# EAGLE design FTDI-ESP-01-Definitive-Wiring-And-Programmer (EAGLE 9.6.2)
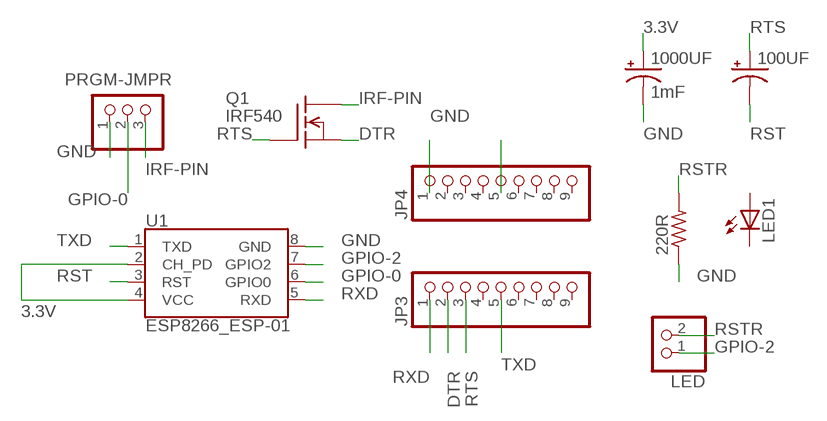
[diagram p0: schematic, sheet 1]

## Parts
100UF  CPOL-USE3.5-8  [E3,5-8]
220R  R-US_0207/2V  [0207/2V]
1000UF  1mF  1000UF-RADIAL-5MM-25V-20%  [CPOL-RADIAL-5MM-10MM]
JP3  PINHD-1X9  [1X09]
JP4  PINHD-1X9  [1X09]
LED  PINHD-1X2  [1X02]
LED1  LED5MM  [LED5MM]
PRGM-JMPR  PINHD-1X3  [1X03]
Q1  IRF540  [TO220]
U1  ESP8266_ESP-01  [ESP8266_ESP-01]

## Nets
3.3V: 1000UF.+ JP4.5 U1.2(CH_PD) U1.4(VCC)
DTR: JP3.2 Q1.3(S)
GND: 220R.1 1000UF.- JP4.1 PRGM-JMPR.1 U1.8(GND)
GPIO-0: PRGM-JMPR.2 U1.6(GPIO0)
GPIO-2: LED.1 U1.7(GPIO2)
IRF-PIN: PRGM-JMPR.3 Q1.2(D)
RST: 100UF.- U1.3(RST)
RSTR: 220R.2 LED.2
RTS: 100UF.+ JP3.3 Q1.1(G)
RXD: JP3.1 U1.5(RXD)
TXD: JP3.5 U1.1(TXD)
Unconnected: JP3.4 JP3.6 JP3.7 JP3.8 JP3.9 JP4.2 JP4.3 JP4.4 JP4.6 JP4.7 JP4.8 JP4.9 LED1.A LED1.K(C)

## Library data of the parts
100UF = adafruit:CPOL-US: POLARIZED CAPACITOR, American symbol
220R = adafruit:R-US_: RESISTOR, American symbol
1000UF = SparkFun-Capacitors:1000UF: 1,000µF/1mF ceramic capacitors; PROD_ID: CAP-09538
JP3 JP4 = pinhead:PINHD-1X9: PIN HEADER
LED = pinhead:PINHD-1X2: PIN HEADER
LED1 = adafruit:LED: LED
PRGM-JMPR = pinhead:PINHD-1X3: PIN HEADER
Q1 = transistor-fet:IRF540: N-Channel Enhancement MOSFET (HEXFET); 100V; 28A; 0,077Ohm
U1 = SparkFun-RF:ESP8266_ESP-01: ESP8266 ESP-01 Module The ESP8266 WiFi Module is a self contained SOC with integrated TCP/IP protocol stack that can give any microcontroller access to your WiFi network. The ESP8266 is capable of either hosting an application or offloading all Wi-Fi networking functions from another application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; SF_ID: WRL-13678

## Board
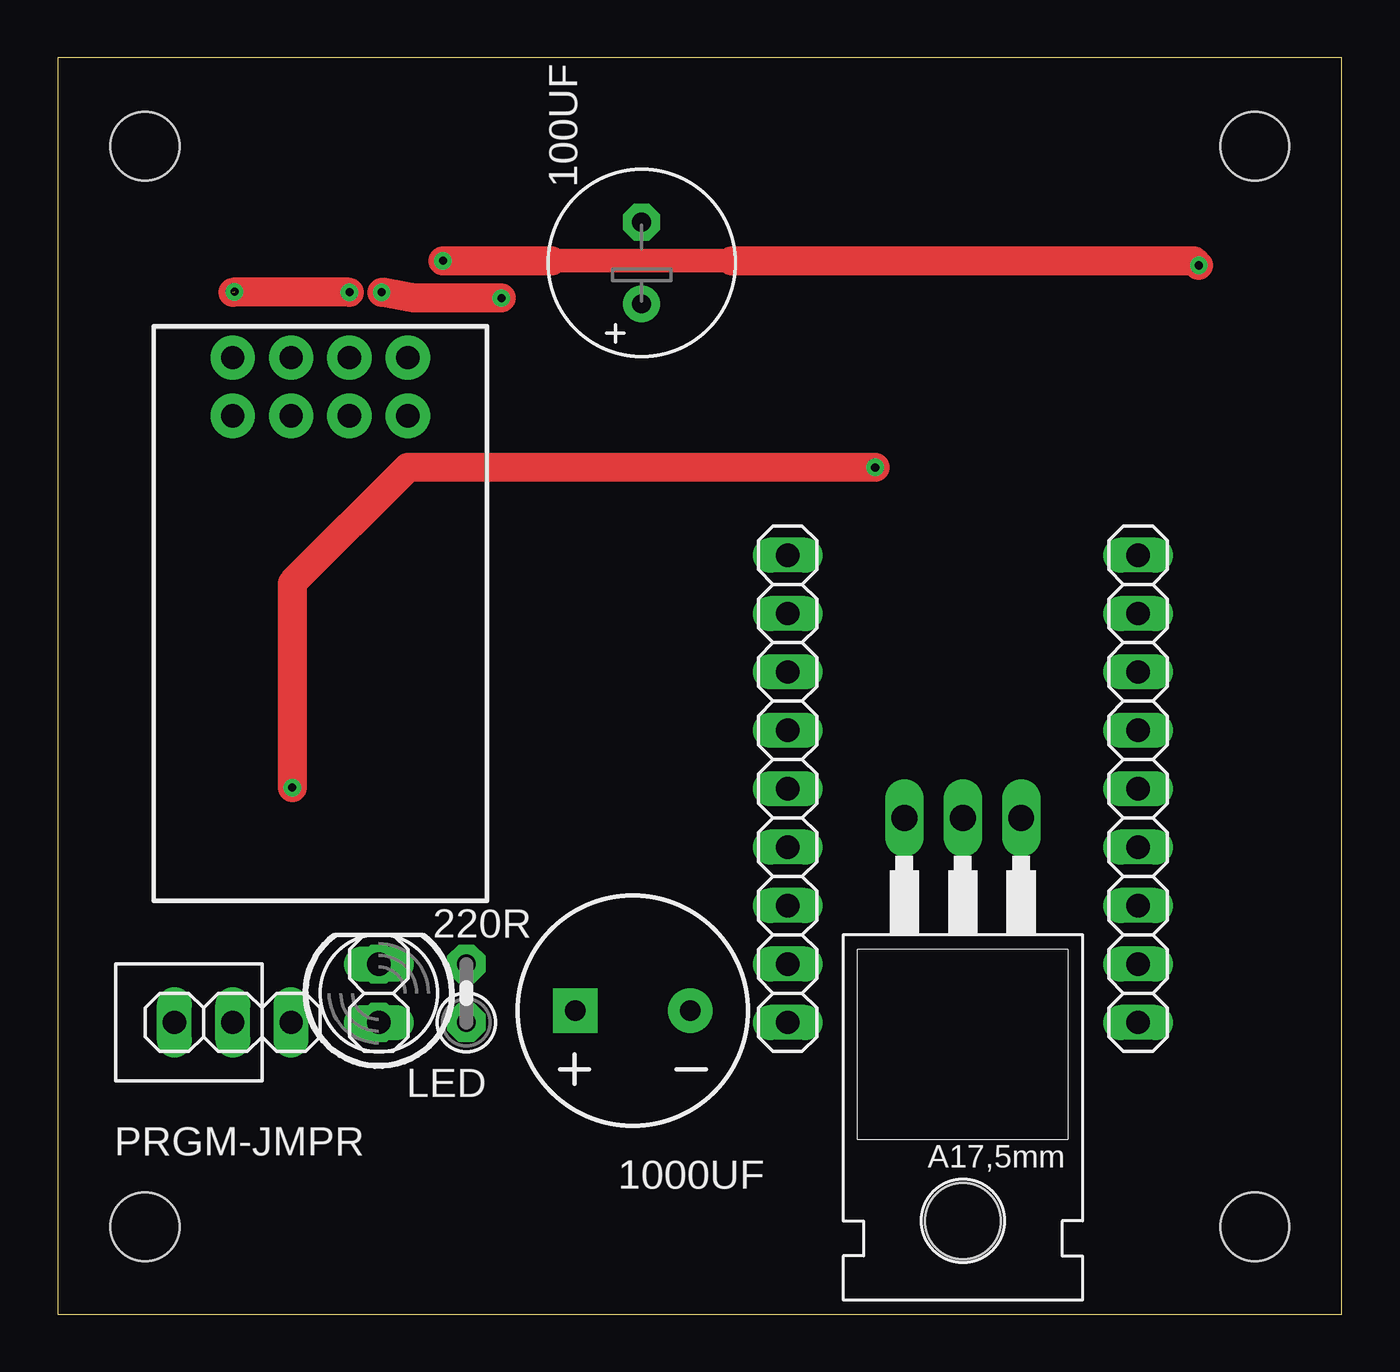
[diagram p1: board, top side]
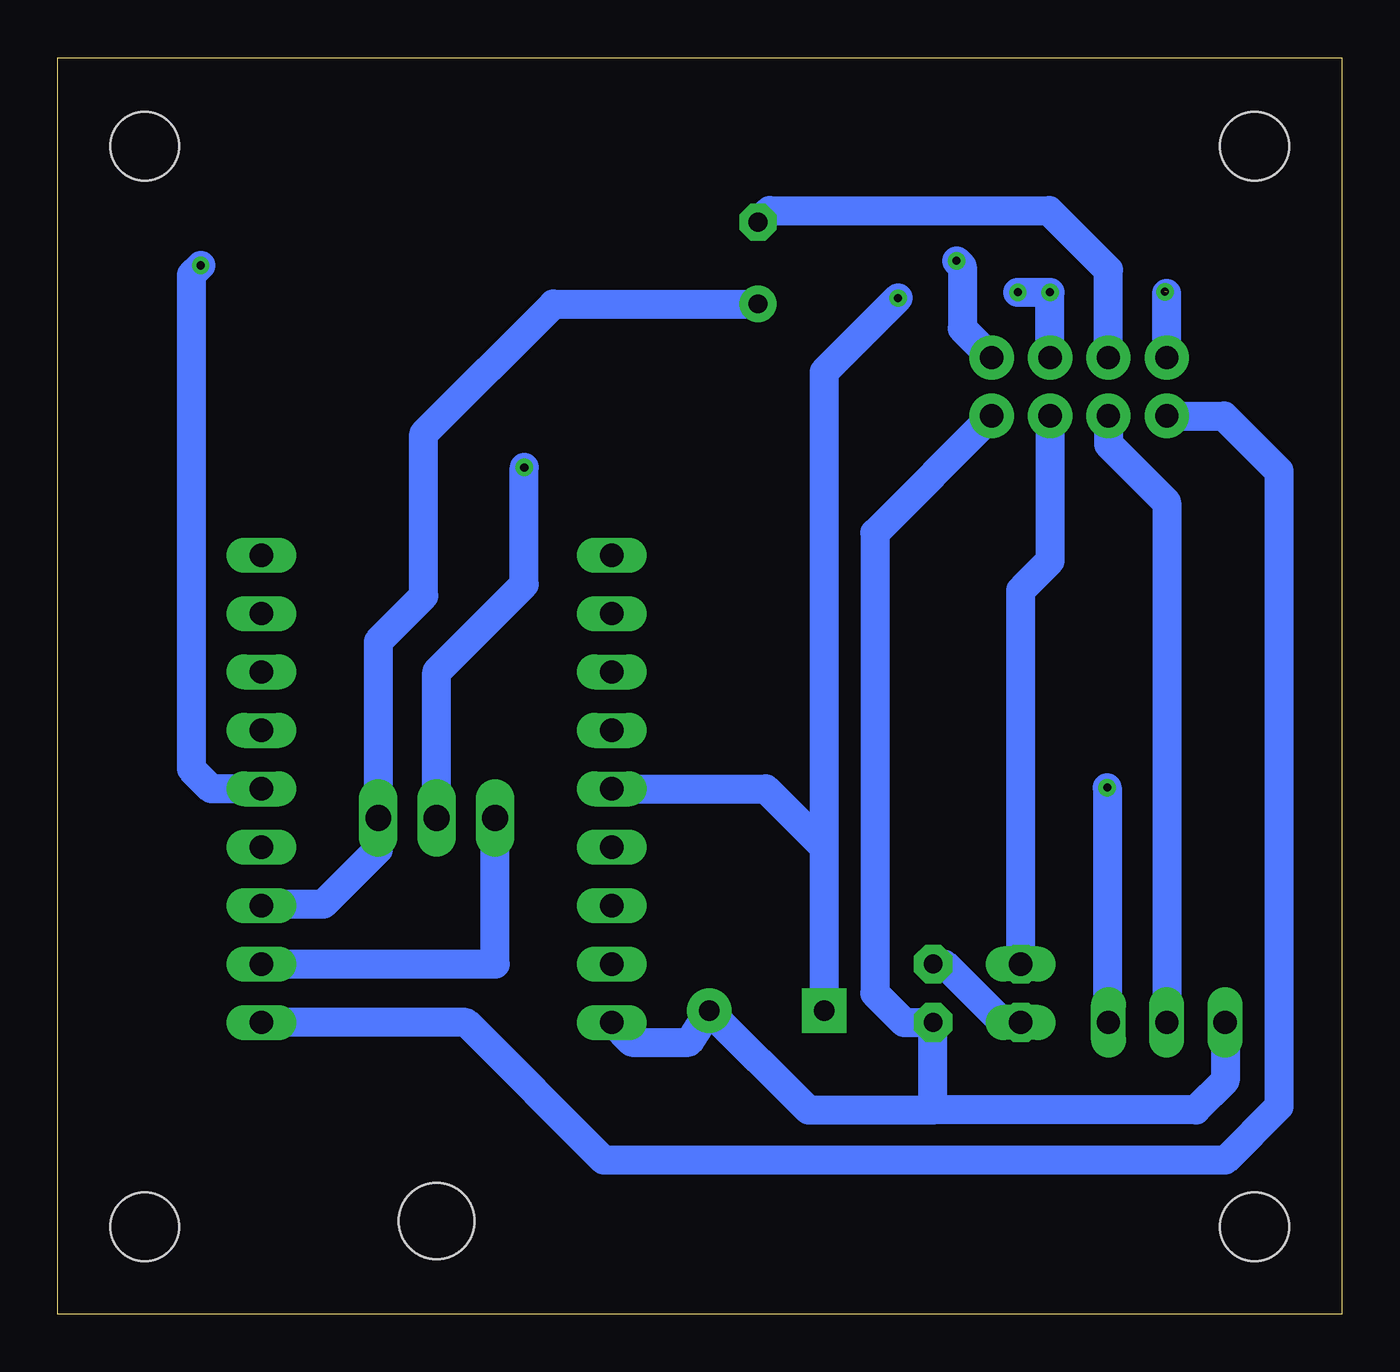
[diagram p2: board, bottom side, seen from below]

Size 55.86 x 54.66 mm. Coordinates in mm from the lower left corner, seen from the top.
Outline: 0,0 55.86,0 55.86,54.66 0,54.66 0,0
Copper layers (1*16): Top 0.035mm / dielectric 1.5mm / Bottom 0.035mm
Design rules "default": minimum track width 6mil, minimum drill 0.35mm, track to track 6mil, track to pad 6mil, pad to pad 6mil, via to via 6mil, smd to smd 6mil, copper to edge 40mil, drill to drill 6mil, minimum pad ring 10mil, minimum via ring 8mil, stop-mask expansion 4mil, vias tented up to drill 0mil, thermal gap 10mil
Holes 3 mm at 3.81,50.8 52.07,50.8 52.07,3.81 3.81,3.81

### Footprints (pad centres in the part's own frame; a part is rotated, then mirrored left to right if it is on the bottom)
E3,5-8 = drill 0.813 pad 1.6: + -1.778,0 | drill 0.813 pad 1.6 octagon: - 1.778,0
0207/2V = drill 0.813 pad 1.676 octagon: 1 -1.27,0; 2 1.27,0
CPOL-RADIAL-5MM-10MM = drill 0.9 pad 1.93 square: + 2.5,0 | drill 0.9 pad 1.93: - -2.5,0
1X09 = drill 1.016 long: 1 -10.16,0; 2 -7.62,0; 3 -5.08,0; 4 -2.54,0; 5 0,0; 6 2.54,0; 7 5.08,0; 8 7.62,0; 9 10.16,0
1X02 = drill 1.016 long: 1 -1.27,0; 2 1.27,0
LED5MM = drill 0.813 pad 1.676 octagon: A -1.27,0; K 1.27,0
1X03 = drill 1.016 long: 1 -2.54,0; 2 0,0; 3 2.54,0
TO220 = drill 1.118 long: 1 -2.54,-6.35; 2 0,-6.35; 3 2.54,-6.35 | hole 3.302: 0,11.176
ESP8266_ESP-01 = drill 1.016 pad 1.93: 1 -3.81,-11.13; 2 -1.27,-11.13; 3 1.27,-11.13; 4 3.81,-11.13; 5 3.81,-8.59; 6 1.27,-8.59; 7 -1.27,-8.59; 8 -3.81,-8.59

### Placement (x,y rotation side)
100UF  25.4,45.72 90 top
220R  17.78,13.97 90 top
1000UF  25.02,13.21 180 top
JP3  46.99,22.86 90 top
JP4  31.75,22.86 90 top
LED  13.97,13.97 270 top
LED1  13.97,13.97 90 top
PRGM-JMPR  7.62,12.7 0 top
Q1  39.37,15.24 180 top
U1  11.43,30.48 180 top

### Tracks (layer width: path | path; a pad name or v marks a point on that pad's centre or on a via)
3.3V  (via drill 0.35)  (1 unrouted)
  Top 1.27: v12.7,44.45 7.62,44.45 | v19.3,44.2 15.49,44.2 v14.1,44.45
  Bottom 0.152: 22.52,20.32 1000UF.+ 22.4,13.11 | 7.62,44.4 v7.7,44.48
  Bottom 1.27: v19.3,44.2 22.52,40.98 1000UF.+ | U1.2 v12.7,44.45 v14.1,44.45 | 22.52,20.32 25.06,22.86 JP4.5 | U1.4 7.62,44.4
DTR
  Bottom 1.27: JP3.2 36.83,15.24 Q1.3
GND
  Bottom 0.152: 17.83,12.8 220R.1 | 15.24,39.17 U1.8
  Bottom 1.27: 5.18,12.65 PRGM-JMPR.1 5.08,10.16 6.35,8.89 17.78,8.89 | JP4.1 30.89,11.84 28.4,11.84 1000UF.- 23.2,8.89 17.78,8.89 | 17.78,8.89 220R.1 19.05,12.7 20.32,13.97 20.32,33.99 U1.8
GPIO-0
  Bottom 1.27: PRGM-JMPR.2 7.62,35.31 10.16,37.85 U1.6
GPIO-2
  Bottom 0.152: 13.97,31.5 13.87,31.6
  Bottom 1.27: 13.87,31.6 12.7,32.77 U1.7 | LED.1 13.97,31.5
IRF-PIN  (via drill 0.35)
  Top 1.27: v35.56,36.83 15.24,36.83 10.21,31.8 v10.21,22.91
  Bottom 0.152: 10.21,12.8 PRGM-JMPR.3
  Bottom 1.27: v10.21,22.91 10.21,12.8 | v35.56,36.83 35.56,31.75 39.37,27.94 Q1.2
RST
  Bottom 1.27: 100UF.- 24.89,48.01 12.75,48.01 10.16,45.42 U1.3
RSTR
  Bottom 0.152: 17.3,15.24 220R.2
  Bottom 1.27: 17.3,15.24 14.86,12.8 14.02,12.8 LED.2
RTS
  Bottom 0.152: 46.94,17.83 JP3.3 | 41.91,20.22 Q1.1
  Bottom 1.27: 46.94,17.83 44.3,17.83 41.91,20.22 | 100UF.+ 34.29,43.94 39.93,38.3 39.93,31.24 41.91,29.26 Q1.1
RXD
  Bottom 1.27: U1.5 5.14,39.07 2.74,36.68 2.74,9.04 5.08,6.71 32.11,6.71 38.1,12.7 JP3.1
TXD  (via drill 0.35)
  Top 0.152: v16.76,45.82 16.77,45.83
  Top 1.016: 21.49,45.82 29.31,45.82
  Top 1.27: v49.63,45.62 49.43,45.82 29.31,45.82 | v16.76,45.82 21.49,45.82
  Bottom 0.152: v49.63,45.62 49.43,45.82
  Bottom 1.27: JP3.5 49.17,22.86 50.04,23.72 50.04,45.21 v49.63,45.62 | v16.76,45.82 16.51,45.57 16.51,42.88 U1.1

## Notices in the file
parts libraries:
SparkFun-RF: Licensing: Creative Commons ShareAlike 4.0 International - https://creativecommons.org/licenses/by-sa/4.0
